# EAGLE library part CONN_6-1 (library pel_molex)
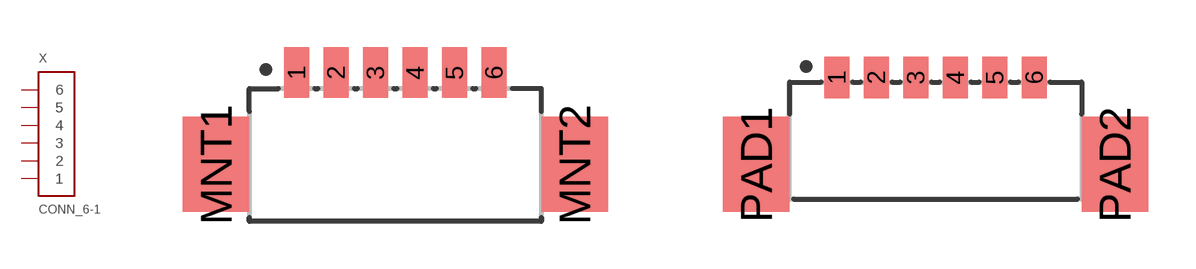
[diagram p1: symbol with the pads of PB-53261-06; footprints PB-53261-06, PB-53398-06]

Designator prefix X

## CONN_6-1-53261  [PB-53261-06]
1  1
2  2
3  3
4  4
5  5
6  6

## CONN_6-1-53398  [PB-53398-06]
Pads as for PB-53261-06

## CONN_6-1-53047  [PB-53047-06]
Pads as for PB-53261-06

## CONN_6-1-502386  [CM-502386-06]
Pads as for PB-53261-06

## CONN_6-1-502382  [CM-502382-06]
Pads as for PB-53261-06

## Footprint PB-53261-06 (pad centres in mm)
smd 0.8 x 1.6: 1 -3.125,1.1; 2 -1.875,1.1; 3 -0.625,1.1; 4 0.625,1.1; 5 1.875,1.1; 6 3.125,1.1
smd 2.1 x 3: MNT1 -5.675,-1.8; MNT2 5.675,-1.8

## Footprint PB-53398-06 (pad centres in mm)
smd 0.8 x 1.3: 1 -3.125,1.25; 2 -1.875,1.25; 3 -0.625,1.25; 4 0.625,1.25; 5 1.875,1.25; 6 3.125,1.25
smd 2.1 x 3: PAD1 -5.675,-1.5; PAD2 5.675,-1.5

## Footprint PB-53047-06 (pad centres in mm)
drill 0.5: 1 -3.125,0; 2 -1.875,0; 3 -0.625,0; 4 0.625,0; 5 1.875,0; 6 3.125,0

## Footprint CM-502386-06 (pad centres in mm)
Click Mate Right Angle
smd 0.6 x 1.7: 1 3.125,-4.55; 2 1.875,-4.55; 3 0.625,-4.55; 4 -0.625,-4.55; 5 -1.875,-4.55; 6 -3.125,-4.55
smd 1 x 2.7: P1 4.975,-1.25; P2 -4.975,-1.25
